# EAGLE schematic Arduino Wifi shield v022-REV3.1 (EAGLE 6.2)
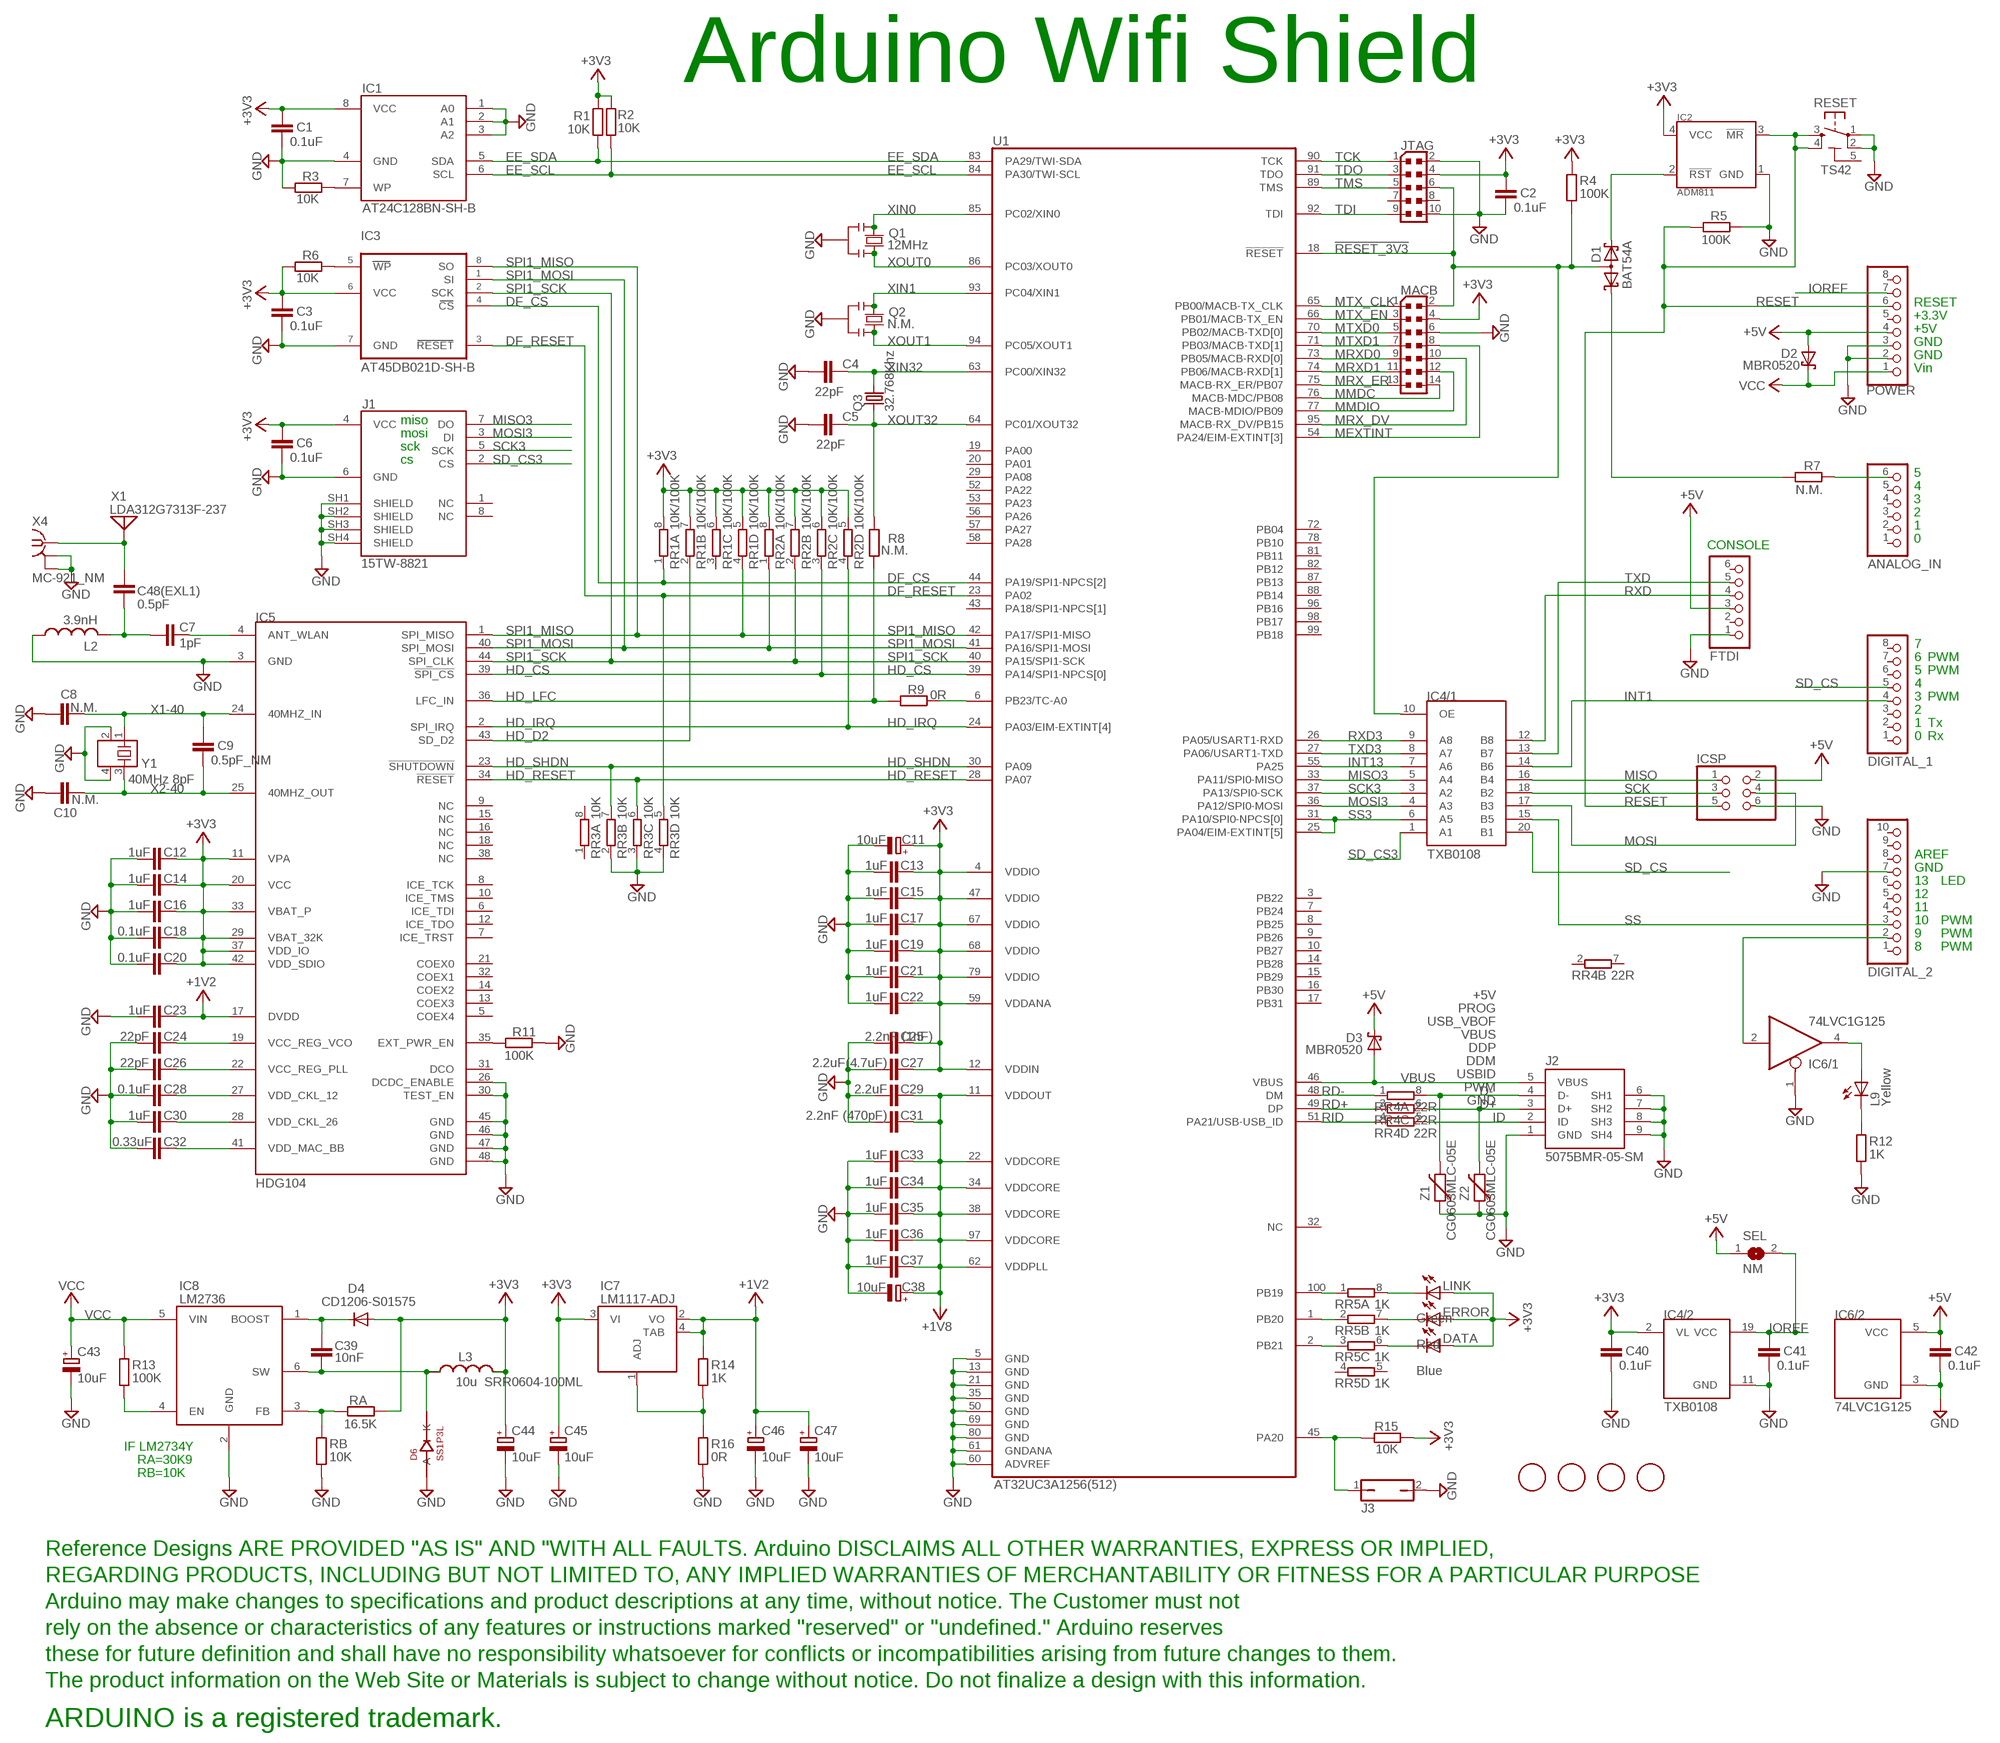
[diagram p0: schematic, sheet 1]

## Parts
ANALOG_IN  PINHD-1X6TH  [1X06-TH]
C1  0.1uF  C-EUC0402  [C0402]
C2  0.1uF  C-EUC0402  [C0402]
C3  0.1uF  C-EUC0402  [C0402]
C4  22pF  C-EUC0402  [C0402]
C5  22pF  C-EUC0402  [C0402]
C6  0.1uF  C-EUC0402  [C0402]
C7  1pF  C-EUC0603K  [C0603K]
C8  N.M.  C-EUC0603  [C0603]
C9  0.5pF_NM  C-EUC0603  [C0603]
C10  N.M.  C-EUC0603  [C0603]
C11  10uF  CPOL-EUSMCB  [SMC_B]
C12  1uF  C-EUC0402  [C0402]
C13  1uF  C-EUC0402  [C0402]
C14  1uF  C-EUC0402  [C0402]
C15  1uF  C-EUC0402  [C0402]
C16  1uF  C-EUC0402  [C0402]
C17  1uF  C-EUC0402  [C0402]
C18  0.1uF  C-EUC0402  [C0402]
C19  1uF  C-EUC0402  [C0402]
C20  0.1uF  C-EUC0402  [C0402]
C21  1uF  C-EUC0402  [C0402]
C22  1uF  C-EUC0402  [C0402]
C23  1uF  C-EUC0402  [C0402]
C24  22pF  C-EUC0603K  [C0603K]
C25  2.2nF (1nF)  C-EUC0603K  [C0603K]
C26  22pF  C-EUC0603K  [C0603K]
C27  2.2uF(4.7uF)  C-EUC0805K  [C0805K]
C28  0.1uF  C-EUC0402  [C0402]
C29  2.2uF  C-EUC0805K  [C0805K]
C30  1uF  C-EUC0402  [C0402]
C31  2.2nF (470pF)  C-EUC0603K  [C0603K]
C32  0.33uF  C-EUC0603K  [C0603K]
C33  1uF  C-EUC0402  [C0402]
C34  1uF  C-EUC0402  [C0402]
C35  1uF  C-EUC0402  [C0402]
C36  1uF  C-EUC0402  [C0402]
C37  1uF  C-EUC0402  [C0402]
C38  10uF  CPOL-EUSMCB  [SMC_B]
C39  10nF  C-EUC0603K  [C0603K]
C40  0.1uF  C-EUC0402  [C0402]
C41  0.1uF  C-EUC0402  [C0402]
C42  0.1uF  C-EUC0402  [C0402]
C43  10uF  CPOL-EUSMCB  [SMC_B]
C44  10uF  CPOL-EUSMCB  [SMC_B]
C45  10uF  CPOL-EUSMCB  [SMC_B]
C46  10uF  CPOL-EUSMCB  [SMC_B]
C47  10uF  CPOL-EUSMCB  [SMC_B]
C48(EXL1)  0.5pF  C-EUC0402  [C0402]
D1  BAT54A  [SOT23]
D2  MBR0520  [DIODE_SOD123]
D3  MBR0520  [DIODE_SOD123]
D4  CD1206-S01575  DIODE-MINIMELF  [MINIMELF]
D6  SS1P3L  [DO220AAL]
DATA  Blue  LEDCHIP-LED0805  [CHIP-LED0805]
DIGITAL_1  PINHD-1X8TH  [1X08-TH]
DIGITAL_2  PINHD-1X10TH  [1X10-TH]
ERROR  Red  LEDCHIP-LED0805  [CHIP-LED0805]
FTDI  PINHD-1X6TH  [1X06-TH]
IC1  AT24C128BN-SH-B  AT24C512B  [SO08]
IC2  ADM811  [ARDUINO_WIFI_SOT143]
IC3  AT45DB021D-SH-B  [8S2]
IC4  TXB0108  [TSSOP20]
IC5  HDG104  [QFN-44-7X7]
IC6  74LVC1G125  74LVC1G125DCK  [74XX-LITTLE-US_SC70-5]
IC7  LM1117-ADJ  [SOT223]
IC8  LM2736  [SOT23-6L]
ICSP  PINHD-2X3  [2X03]
J1  15TW-8821  SDCARD-15TW-8821-SPI  [SDCARD-15TW-8821]
J2  5075BMR-05-SM  USB-MINI-B%C  [USB-MINI-B_2]
J3  JP1Q  [JP1]
JTAG  PINHEAD_PINHD-2X5PASSO127  [PINHEAD_2X05_127]
L2  3.9nH  L-USL0402  [L0402]
L3  10u SRR0604-100ML  L-USSRR0604  [SRR0604]
L9  Yellow  LEDCHIP-LED0805  [CHIP-LED0805]
LINK  Green  LEDCHIP-LED0805  [CHIP-LED0805]
MACB  PINHEAD_PINHD-2X7PASSO127  [PINHEAD_2X07_127]
POWER  PINHD-1X8TH  [1X08-TH]
Q1  12MHz  SMD_RESONATORMU  [SMD_RESONATOR]
Q2  N.M.  SMD_RESONATORMU  [SMD_RESONATOR]
Q3  32.768Khz  RESONATOR_EPSON_FC_145  [RESONATOR_EPSON_FC_145]
R1  10K  R-EU_R0402  [R0402]
R2  10K  R-EU_R0402  [R0402]
R3  10K  R-EU_R0402  [R0402]
R4  100K  R-EU_R0402  [R0402]
R5  100K  R-EU_R0402  [R0402]
R6  10K  R-EU_R0402  [R0402]
R7  N.M.  R-EU_R0402  [R0402]
R8  N.M.  R-EU_R0402  [R0402]
R9  0R  R-EU_R0402  [R0402]
R11  100K  R-EU_R0402  [R0402]
R12  1K  R-EU_R0402  [R0402]
R13  100K  R-EU_R0402  [R0402]
R14  1K  R-EU_R0603  [R0603]
R15  10K  R-EU_R0402  [R0402]
R16  0R  R-EU_R0402  [R0402]
RA  16.5K  R-EU_R0603  [R0603]
RB  10K  R-EU_R0603  [R0603]
RESET  TS42  ST-MOD_V1.4_TS42  [ST-MOD_V1.4_TS42]
RR1  10K/100K  4R-NCAY16  [CAY16]
RR2  10K/100K  4R-NCAY16  [CAY16]
RR3  10K  4R-NCAY16  [CAY16]
RR4  22R  4R-NCAY16  [CAY16]
RR5  1K  4R-NCAY16  [CAY16]
SEL  NM  SJL  [SJL]
U1  AT32UC3A1256(512)  AT32UC3A1512  [TQFP100]
U$1  FIDUCIALMOUNT  [FIDUCIA-MOUNT]
U$2  FIDUCIALMOUNT  [FIDUCIA-MOUNT]
U$3  FIDUCIALMOUNT  [FIDUCIA-MOUNT]
U$4  FIDUCIALMOUNT  [FIDUCIA-MOUNT]
U$5  DISCLAIMER  [DISCLAIMER]
X1  LDA312G7313F-237  [LDA31]
X4  MC-921_NM  MC-921  [MC-921]
Y1  40MHz 8pF  ABM10  [ARDUINO_WIFI_2.5X2.0]
Z1  CG0603MLC-05E  VARISTORCN0603  [CT/CN0603]
Z2  CG0603MLC-05E  VARISTORCN0603  [CT/CN0603]

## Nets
!RESET_3V3: D1.3(AA) IC4.10(/1:OE) JTAG.6 MACB.2 R4.2 U1.18(!RESET)
+1V2: C23.1 C46.+ C47.+ IC5.17(DVDD) IC7.2(VO) IC7.4(TAB) R14.2
+1V8: C29.1 C31.1 C33.1 C34.1 C35.1 C36.1 C37.1 C38.+ U1.11(VDDOUT) U1.22(VDDCORE) U1.34(VDDCORE) U1.38(VDDCORE) U1.62(VDDPLL) U1.97(VDDCORE)
+3V3: C1.1 C2.1 C3.1 C6.1 C11.+ C12.1 C13.1 C14.1 C15.1 C16.1 C17.1 C18.1 C19.1 C20.1 C21.1 C22.1 C25.1 C27.1 C40.1 C44.+ C45.+ D4.A DATA.A ERROR.A IC1.8(VCC) IC2.4(VCC) IC3.P$6(VCC) IC4.2(/2:VL) IC5.11(VPA) IC5.20(VCC) IC5.29(VBAT_32K) IC5.33(VBAT_P) IC5.37(VDD_IO) IC5.42(VDD_SDIO) IC7.3(VI) J1.4(VCC) JTAG.4 L3.P$2 LINK.A MACB.4 R1.1 R2.1 R4.1 R6.2 R15.1 RA.1 RR1.5 RR1.6 RR1.7 RR1.8 RR2.5 RR2.6 RR2.7 RR2.8 U1.4(VDDIO) U1.12(VDDIN) U1.47(VDDIO) U1.59(VDDANA) U1.67(VDDIO) U1.68(VDDIO) U1.79(VDDIO)
+5V: C42.1 D2.A D3.C FTDI.3 IC6.5(/2:VCC) ICSP.2 POWER.4 SEL.1
D+: J2.3(D+) RR4.6 Z2.2
D-: J2.4(D-) RR4.8 Z1.2
DF_CS: IC3.P$4(CS) RR1.1 U1.44(PA19/SPI1-NPCS[2])
DF_RESET: IC3.P$3(RESET) RR3.5 U1.23(PA02)
EE_SCL: IC1.6(SCL) R2.2 U1.84(PA30/TWI-SCL)
EE_SDA: IC1.5(SDA) R1.2 U1.83(PA29/TWI-SDA)
GND: C1.2 C2.2 C3.2 C4.1 C5.1 C6.2 C8.1 C10.1 C11.- C12.2 C13.2 C14.2 C15.2 C16.2 C17.2 C18.2 C19.2 C20.2 C21.2 C22.2 C23.2 C24.2 C25.2 C26.2 C27.2 C28.2 C29.2 C30.2 C31.2 C32.2 C33.2 C34.2 C35.2 C36.2 C37.2 C38.- C40.2 C41.2 C42.2 C43.- C44.- C45.- C46.- C47.- D6.P$2(A) DIGITAL_2.7 FTDI.1 IC1.1(A0) IC1.2(A1) IC1.3(A2) IC1.4(GND) IC2.1(GND) IC3.P$7(GND) IC4.11(/2:GND) IC5.3(GND) IC5.26(DCDC_ENABLE) IC5.30(TEST_EN) IC5.45(GND) IC5.46(GND) IC5.47(GND) IC5.48(GND) IC6.1(/1:OE) IC6.3(/2:GND) IC8.2(GND) ICSP.6 J1.6(GND) J1.SH1(SHIELD) J1.SH2(SHIELD) J1.SH3(SHIELD) J1.SH4(SHIELD) J2.1(GND) J2.6(SH1) J2.7(SH2) J2.8(SH3) J2.9(SH4) J3.2 JTAG.2 JTAG.10 L2.1 MACB.6 POWER.2 POWER.3 Q1.2 Q2.2 R3.2 R5.1 R11.2 R12.2 R16.1 RB.1 RESET.1 RESET.2 RR3.2 RR3.3 RR3.4 U1.5(GND) U1.13(GND) U1.21(GND) U1.35(GND) U1.50(GND) U1.60(ADVREF) U1.61(GNDANA) U1.69(GND) U1.80(GND) X4.2@1(GND) X4.2@2(GND) Y1.2 Y1.4 Z1.1 Z2.1
HD_CS: IC5.39(!SPI_CS) RR2.3 U1.39(PA14/SPI1-NPCS[0])
HD_D2: IC5.43(SD_D2) RR1.2
HD_IRQ: IC5.2(SPI_IRQ) RR2.4 U1.24(PA03/EIM-EXTINT[4])
HD_LFC: IC5.36(LFC_IN) R8.2 R9.2
HD_RESET: IC5.34(!RESET) RR3.6 U1.28(PA07)
HD_SHDN: IC5.23(!SHUTDOWN) RR3.7 U1.30(PA09)
ID: J2.2(ID) RR4.5
INT1: DIGITAL_1.4 IC4.14(/1:B6)
INT13: IC4.7(/1:A6) U1.55(PA25)
IOREF: C41.1 IC4.19(/2:VCC) POWER.7 SEL.2
MEXTINT: MACB.8 U1.54(PA24/EIM-EXTINT[3])
MISO: IC4.16(/1:B4) ICSP.1
MISO3: IC4.5(/1:A4) J1.7(DO) U1.33(PA11/SPI0-MISO)
MMDC: MACB.14 U1.76(MACB-MDC/PB08)
MMDIO: MACB.12 U1.77(MACB-MDIO/PB09)
MOSI: IC4.17(/1:B3) ICSP.4
MOSI3: IC4.4(/1:A3) J1.3(DI) U1.36(PA12/SPI0-MOSI)
MRX_DV: MACB.10 U1.95(MACB-RX_DV/PB15)
MRX_ER: MACB.13 U1.75(MACB-RX_ER/PB07)
MRXD0: MACB.9 U1.73(PB05/MACB-RXD[0])
MRXD1: MACB.11 U1.74(PB06/MACB-RXD[1])
MTX_CLK: MACB.1 U1.65(PB00/MACB-TX_CLK)
MTX_EN: MACB.3 U1.66(PB01/MACB-TX_EN)
MTXD0: MACB.5 U1.70(PB02/MACB-TXD[0])
MTXD1: MACB.7 U1.71(PB03/MACB-TXD[1])
N$1: IC3.P$5(WP) R6.1
N$2: R9.1 U1.6(PB23/TC-A0)
N$3: DIGITAL_2.2 IC6.2(/1:I)
N$4: C24.1 IC5.19(VCC_REG_VCO)
N$5: D1.2(K2) IC2.2(!RST)
N$6: C26.1 IC5.22(VCC_REG_PLL)
N$7: IC8.3(FB) RA.2 RB.2
N$8: IC1.7(WP) R3.1
N$10: IC7.1(ADJ) R14.1 R16.2
N$17: IC8.4(EN) R13.1
N$18: C39.1 D4.C IC8.1(BOOST)
N$20: C28.1 IC5.27(VDD_CKL_12)
N$31: C30.1 IC5.28(VDD_CKL_26)
N$32: C32.1 IC5.41(VDD_MAC_BB)
N$33: C7.2 C48(EXL1).2 L2.2
N$34: IC5.35(EXT_PWR_EN) R11.1
N$39: IC6.4(/1:O) L9.A
N$40: C39.2 D6.P$1(K) IC8.6(SW) L3.P$1
N$46: ANALOG_IN.6 R7.1
N$49: D1.1(K1) R7.2
N$52: LINK.C RR5.8
N$53: ERROR.C RR5.7
N$54: DATA.C RR5.6
N$55: L9.C R12.1
N$56: RR5.1 U1.100(PB19)
N$57: RR5.2 U1.1(PB20)
N$58: C7.1 IC5.4(ANT_WLAN)
N$59: C48(EXL1).1 X1.1 X4.1
N$60: RR5.3 U1.2(PB21)
N$61: J3.1 R15.2 U1.45(PA20)
RD+: RR4.3 U1.49(DP)
RD-: RR4.1 U1.48(DM)
RESET: IC2.3(!MR) ICSP.5 POWER.6 R5.2 RESET.3 RESET.4
RID: RR4.4 U1.51(PA21/USB-USB_ID)
RXD: FTDI.4 IC4.12(/1:B8)
RXD3: IC4.9(/1:A8) U1.26(PA05/USART1-RXD)
SCK: IC4.18(/1:B2) ICSP.3
SCK3: IC4.3(/1:A2) J1.5(SCK) U1.37(PA13/SPI0-SCK)
SD_CS: DIGITAL_1.5 IC4.20(/1:B1)
SD_CS3: IC4.1(/1:A1) J1.2(CS)
SPI1_MISO: IC3.P$8(SO) IC5.1(SPI_MISO) RR1.4 U1.42(PA17/SPI1-MISO)
SPI1_MOSI: IC3.P$1(SI) IC5.40(SPI_MOSI) RR2.1 U1.41(PA16/SPI1-MOSI)
SPI1_SCK: IC3.P$2(SCK) IC5.44(SPI_CLK) RR2.2 U1.40(PA15/SPI1-SCK)
SS: DIGITAL_2.3 IC4.15(/1:B5)
SS3: IC4.6(/1:A5) U1.25(PA04/EIM-EXTINT[5]) U1.31(PA10/SPI0-NPCS[0])
TCK: JTAG.1 U1.90(TCK)
TDI: JTAG.9 U1.92(TDI)
TDO: JTAG.3 U1.91(TDO)
TMS: JTAG.5 U1.89(TMS)
TXD: FTDI.5 IC4.13(/1:B7)
TXD3: IC4.8(/1:A7) U1.27(PA06/USART1-TXD)
VBUS: D3.A J2.5(VBUS) U1.46(VBUS)
VCC: C43.+ D2.C IC8.5(VIN) POWER.1 R13.2
X1-40: C8.2 C9.1 IC5.24(40MHZ_IN) Y1.1
X2-40: C9.2 C10.2 IC5.25(40MHZ_OUT) Y1.3
XIN0: Q1.1 U1.85(PC02/XIN0)
XIN1: Q2.1 U1.93(PC04/XIN1)
XIN32: C4.2 Q3.P$2 U1.63(PC00/XIN32)
XOUT0: Q1.3 U1.86(PC03/XOUT0)
XOUT1: Q2.3 U1.94(PC05/XOUT1)
XOUT32: C5.2 Q3.P$1 R8.1 U1.64(PC01/XOUT32)
Unconnected: ANALOG_IN.1 ANALOG_IN.2 ANALOG_IN.3 ANALOG_IN.4 ANALOG_IN.5 DIGITAL_1.1 DIGITAL_1.2 DIGITAL_1.3 DIGITAL_1.6 DIGITAL_1.7 DIGITAL_1.8 DIGITAL_2.1 DIGITAL_2.4 DIGITAL_2.5 DIGITAL_2.6 DIGITAL_2.8 DIGITAL_2.9 DIGITAL_2.10 FTDI.2 FTDI.6 IC5.5(COEX4) IC5.6(ICE_TDI) IC5.7(ICE_TRST) IC5.8(ICE_TCK) IC5.9(NC) IC5.10(ICE_TMS) IC5.12(ICE_TDO) IC5.13(COEX3) IC5.14(COEX2) IC5.15(NC) IC5.16(NC) IC5.18(NC) IC5.21(COEX0) IC5.31(DCO) IC5.32(COEX1) IC5.38(NC) J1.1(NC) J1.8(NC) JTAG.7 JTAG.8 POWER.5 POWER.8 RESET.5(5-GND) RR1.3 RR3.1 RR3.8 RR4.2 RR4.7 RR5.4 RR5.5 U1.3(PB22) U1.7(PB24) U1.8(PB25) U1.9(PB26) U1.10(PB27) U1.14(PB28) U1.15(PB29) U1.16(PB30) U1.17(PB31) U1.19(PA00) U1.20(PA01) U1.29(PA08) U1.32(NC) U1.43(PA18/SPI1-NPCS[1]) U1.52(PA22) U1.53(PA23) U1.56(PA26) U1.57(PA27) U1.58(PA28) U1.72(PB04) U1.78(PB10) U1.81(PB11) U1.82(PB12) U1.87(PB13) U1.88(PB14) U1.96(PB16) U1.98(PB17) U1.99(PB18)

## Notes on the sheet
- Arduino Wifi Shield
- RESET
- +3.3V
- +5V
- GND
- GND
- Vin
- miso
- mosi
- sck
- cs
- 5
- 4
- 3
- 2
- 1
- 0
- CONSOLE
- 7
- 6 | PWM
- 5 | PWM
- 4
- 3 | PWM
- 2
- 1 | Tx
- 0 | Rx
- AREF
- GND
- 13 | LED
- 12
- 11
- 10 | PWM
- 9 | PWM
- 8 | PWM
- +5V
- PROG
- USB_VBOF
- VBUS
- DDP
- DDM
- USBID
- PWM
- GND
- IF LM2734Y
- RA=30K9
- RB=10K

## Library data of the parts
ANALOG_IN FTDI = SmartPrj:PINHD-1X6: PIN HEADER
C1 C3 C6 C8 C10 C42 = rcl:C-EU: CAPACITOR, European symbol
C2 C4 C5 C7 C9 C12-C14 C16-C26 C28 C30-C32 C34-C37 C39-C41 C48(EXL1) = Arduino_Wifi_shield_v018_tG:C-EU: CAPACITOR, European symbol
C11 C38 C43-C47 = rcl:CPOL-EU: POLARIZED CAPACITOR, European symbol
C15 C27 C29 C33 = resistor:C-EU: CAPACITOR, European symbol
D1 = diode:BAT54A: Schottky Diodes Source: Fairchild .. BAT54.pdf
D2 D3 = arduino_wifi:MBR0520
D4 = diode:DIODE-: DIODE
D6 = SmartPrj:SS1P3L
DATA ERROR L9 LINK = led:LED: LED
DIGITAL_1 POWER = SmartPrj:PINHD-1X8: PIN HEADER
DIGITAL_2 = SmartPrj:PINHD-1X10: PIN HEADER
IC1 = Arduino_Wifi_shield_v018_tG:AT24C512B
IC2 = arduino_wifi:ADM811
IC3 = SmartPrj:AT45DB021D-SH-B: AT45DB021D-SH B
IC4 = Arduino_Wifi_shield_v018_tG:TXB0108
IC5 = arduino_wifi:HDG104
IC6 = arduino_wifi:74LVC1G125
IC7 = arduino_wifi:LM1117-ADJ: LM1117-ADJ. Linear adjustable regulator. National Semiconductor
IC8 = arduino_wifi:LM2736: 750mA Load Step-Down DC-DC Regulator. National Semiconductor.
ICSP = SmartPrj:PINHD-2X3: PIN HEADER
J1 = arduino_wifi:SDCARD-15TW-8821-SPI
J2 = MyCON2:USB-MINI-B
J3 = jumper:JP1Q: JUMPER
JTAG = Arduino_Wifi_shield_v018_tG:PINHEAD_PINHD-2X5: PIN HEADER
L2 = rcl-2:L-US: INDUCTOR, American symbol
L3 = SmartPrj:L-US: INDUCTOR, American symbol
MACB = Arduino_Wifi_shield_v018_tG:PINHEAD_PINHD-2X7: PIN HEADER
Q1 Q2 = SmartPrj:SMD_RESONATOR
Q3 = Arduino_Wifi_shield_v018_tG:RESONATOR_EPSON_FC_145
R1-R4 R6 R8 R9 R11 RA RB = Arduino_Wifi_shield_v018_tG:R-EU_: RESISTOR, European symbol
R5 R7 R12 R14-R16 = resistor:R-EU_: RESISTOR, European symbol
R13 = rcl:R-EU_: RESISTOR, European symbol
RESET = Arduino_Wifi_shield_v018_tG:ST-MOD_V1.4_TS42: TS42 Dongnan Electronics Tact switch VDC 12V - 50mA
RR1-RR5 = resistor-dil:4R-N: Array Chip Resistor Source: RS Component / Phycomp
SEL = SmartPrj:SJ: SMD solder JUMPER
U1 = Arduino_Wifi_shield_v018_tG:AT32UC3A1512: AT32UC3A1512/1256/1128
U$1-U$4 = SmartPrj:FIDUCIALMOUNT
U$5 = SmartPrj:DISCLAIMER
X1 = Arduino wifi:LDA312G7313F-237
X4 = con-coax:MC-921: COAX. MICROWAVE CONNECTOR O/D diam 2.1 Source: www.tycoelectronics.com .. Electronics .. ENG_CD_1775146_A2.pdf; OC_FARNELL: unknown; OC_NEWARK: unknown
Y1 = arduino_wifi:ABM10
Z1 Z2 = varistor:VARISTOR: VARISTOR

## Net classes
0 default: width 0.203 mm, drill 0.305 mm, clearance 0.178 mm
1 power: width 0.254 mm, drill 0.61 mm, clearance 0.203 mm
2 VIN: width 0.61 mm, drill 0.813 mm, clearance 0.305 mm
3 usbvcc: width 0.508 mm, drill 0.508 mm, clearance 0.152 mm
4 aref: width 0.406 mm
